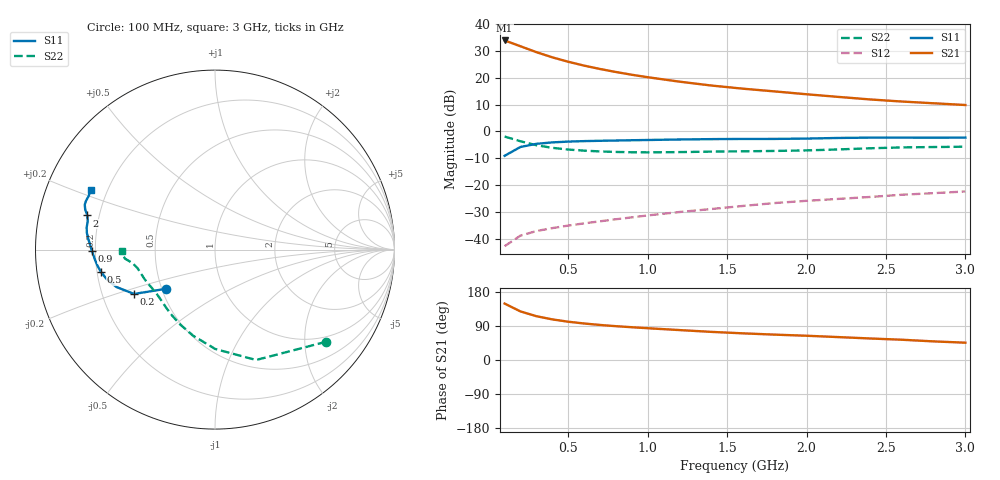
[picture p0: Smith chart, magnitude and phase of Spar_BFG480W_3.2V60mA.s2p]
! Filename: 3_260BFG480.001
! Title: BFG480W
! Bias: Vce=3.2V; Ic=60mA
! Company: NXP Semiconductors NL
! User: Quality&Reliability T&D
! Measure time: 10 Nov 1999 / 11:57:10
#  MHz  S  MA  R 50
! Freq  S11  S21  S12  S22  :
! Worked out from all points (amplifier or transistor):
!   20 points, 100 MHz to 3 GHz, reference 50 ohm
!   highest |S21| = 33.9 dB at 100 MHz (marker M1)
!   |S21| within 3 dB of that: start of sweep to 238 MHz
!   unconditionally stable (mu >= 1): 881.4 MHz to end of sweep
!   at 400 MHz: K = 0.70, MSG = 31.8 dB, |S12| = -36.0 dB
!   at 1.2 GHz: K = 1.06, MAG = 22.8 dB, |S12| = -30.0 dB
!   at 3 GHz: K = 1.06, MAG = 14.6 dB, |S12| = -22.4 dB
!   S11 on the Smith chart (normalised r, x): 100 MHz: 0.52, -0.26; 200 MHz: 0.34, -0.23; 500 MHz: 0.22, -0.09; 900 MHz: 0.19, -0.00; 2 GHz: 0.15, +0.13; 3 GHz: 0.14, +0.22
100  0.3516 -141.5  49.81 148.9  0.007262 68.9  0.8045 -39.7
200  0.5144 -151.3  38.82 128.2  0.01143 58.2  0.6563 -69.6
300  0.5883 -159.3  30.15 115.6  0.01388 55.2  0.5538 -89.8
400  0.6256 -164.8  24.14 107.2  0.01577 55.4  0.4951 -104.2
500  0.6473 -168.9  19.98 101.0  0.01757 56.8  0.4604 -114.8
600  0.661 -172.2  16.92 96.3  0.01931 58.6  0.4389 -122.8
700  0.6701 -174.9  14.64 92.5  0.02111 60.7  0.4246 -129.1
800  0.6778 -177.3  12.86 89.3  0.02307 62.8  0.4152 -134.3
900  0.6864 -179.5  11.43 86.5  0.02499 64.7  0.4098 -138.8
1000  0.6935 178.5  10.29 83.9  0.02718 66.2  0.4079 -142.9
1200  0.7087 175.1  8.497 79.0  0.03146 68.4  0.4124 -149.4
1400  0.7199 172.6  7.198 74.2  0.03578 70.1  0.4212 -154.4
1600  0.7258 170.1  6.28 70.3  0.04085 71.4  0.4267 -158.1
1800  0.7264 167.4  5.585 67.0  0.04629 72.4  0.4333 -162.0
2000  0.7368 165.0  4.944 64.0  0.05091 73.4  0.4436 -166.4
2200  0.7571 162.8  4.414 60.5  0.05527 73.6  0.4622 -170.2
2400  0.7677 161.0  3.956 56.8  0.06008 73.4  0.486 -172.7
2600  0.7683 159.2  3.618 53.5  0.06607 72.9  0.5043 -174.3
2800  0.7645 157.0  3.356 49.1  0.07076 71.7  0.5127 -176.2
3000  0.7695 154.3  3.116 45.7  0.07607 71.1  0.5201 -179.2
